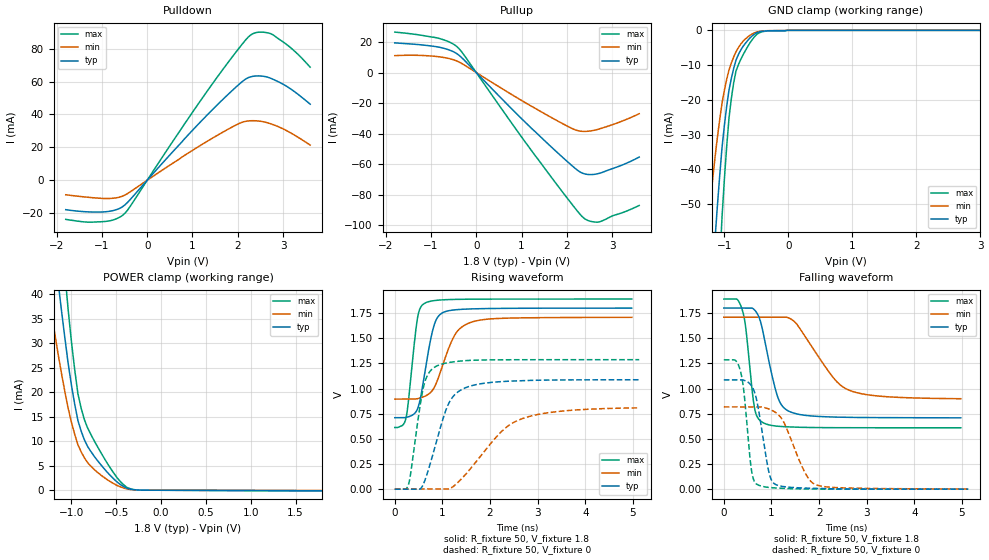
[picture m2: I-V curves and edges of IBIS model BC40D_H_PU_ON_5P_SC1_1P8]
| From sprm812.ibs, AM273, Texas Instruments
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|   Model Cell BC40D_H_PU_ON_5P_SC1_1P8
|BC40D_H_PU_ON_5P_SC1_1P8
[Model]   BC40D_H_PU_ON_5P_SC1_1P8
Model_type   I/O
Polarity   Non-Inverting
Enable   Active-Low
Vinl =  0.63
Vinh =  1.17
Cref =  15pF
Rref =  100.0000M
Vref =  0V
Vmeas =  0.9
C_comp   2.364487p   2.290698p   2.389419p
|[Input load] weak_pu_on
|[Output drive] slow
|[supplytol] 5
|[temp] ind
[Model Spec]
Vinl   0.63   0.5985   0.6615
Vinh   1.17   1.1115   1.2285
[Temperature Range]   25   125   -40
[Voltage Range]   1.8   1.71   1.89
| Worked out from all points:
|   slope of the pulldown table from 0 to 0.27 V, typ, clamps not added: 32.2 ohm
|   slope of the pullup table from 0 to 0.27 V, typ, clamps not added: 32.6 ohm
|   GND clamp passes 1 mA (typ) near -0.52 V on its own axis
|   POWER clamp passes 1 mA (typ) near -0.44 V on its own axis
|   rising waveform, R_fixture 50, V_fixture 1.8: 20-80 % time 249ps typ, 402ps min, 171ps max; typ from 0.71 V to 1.8 V
|   rising waveform, R_fixture 50, V_fixture 0: 20-80 % time 430ps typ, 919ps min, 246ps max; typ from 0 V to 1.09 V
|   falling waveform, R_fixture 50, V_fixture 1.8: 20-80 % time 310ps typ, 721ps min, 172ps max; typ from 1.8 V to 0.71 V
|   falling waveform, R_fixture 50, V_fixture 0: 20-80 % time 228ps typ, 434ps min, 155ps max; typ from 1.09 V to 0.002 V
| Nom Voltages:
|   VDD=1.1, VDDS=1.8, VDDS18=1.8, ESD_BIASFET=0, VSS=0, VSSS=0
| Min Voltages:
|   VDD=1.045, VDDS=1.71, VDDS18=1.71, ESD_BIASFET=0, VSS=0, VSSS=0
| Max Voltages:
|   VDD=1.16, VDDS=1.89, VDDS18=1.89, ESD_BIASFET=0, VSS=0, VSSS=0
[POWER_clamp]
|   voltage   I(typ)   I(min)   I(max)
-1.8V     158.8mA    112.5mA    219.8mA
-1.255V   59.97mA    40.01mA    84.91mA
-1.145V   41.92mA    27.41mA    59.76mA
-1.109V   36.32mA    23.62mA    51.83mA
-1.073V   30.96mA    20.04mA    44.16mA
-1.036V   25.83mA    16.67mA    36.76mA
-963.6mV  17.54mA    11.39mA    24.56mA
-890.9mV  12.01mA    7.798mA    16.67mA
-818.2mV  8.875mA    5.598mA    12.64mA
-563.6mV  2.954mA    1.726mA    4.46mA
-272.7mV  55.97uA    39.54uA    57.56uA
1.8V      -99.94uA   -59.14uA   -145.1uA
[Pulldown]
|   voltage   I(typ)   I(min)   I(max)
-1.8V     -17.92mA   -8.85mA    -23.8mA
-1.309V   -19.26mA   -10.37mA   -25.51mA
-927.3mV  -19.22mA   -11.12mA   -25.08mA
-654.5mV  -17.65mA   -10.56mA   -23.13mA
-490.9mV  -14.97mA   -8.985mA   -20.05mA
1.364V    40.78mA    24.32mA    55.7mA
2.073V    59.41mA    35mA       81.9mA
2.291V    62.96mA    36.2mA     88.48mA
2.509V    63.41mA    35.84mA    90.12mA
2.782V    61.38mA    33.82mA    88.42mA
3.218V    54.59mA    28.02mA    79.45mA
3.6V      46.26mA    21.39mA    68.79mA
[Pullup]
|   voltage   I(typ)   I(min)   I(max)
-1.8V     19.42mA    11.07mA    26.5mA
-818.2mV  16.58mA    10.3mA     22.34mA
-545.5mV  14.19mA    8.748mA    19.29mA
-381.8mV  11.34mA    6.915mA    15.7mA
1.255V    -37.51mA   -22.64mA   -52.53mA
2.127V    -61.34mA   -36.82mA   -86.78mA
2.291V    -65.12mA   -38.38mA   -92.82mA
2.4V      -66.46mA   -38.59mA   -95.91mA
2.564V    -66.86mA   -38.08mA   -97.75mA
2.727V    -65.99mA   -36.9mA    -97.78mA
3.273V    -60.01mA   -31.26mA   -91.34mA
3.6V      -55.4mA    -26.98mA   -87.12mA
[GND_clamp]
|   voltage   I(typ)   I(min)   I(max)
-1.8V     -270.2mA   -170.2mA   -430.1mA
-1.255V   -91.68mA   -55.92mA   -148.5mA
-1.145V   -59.94mA   -36.46mA   -97.14mA
-1.109V   -50.51mA   -30.84mA   -81.61mA
-1.073V   -41.77mA   -25.67mA   -67.13mA
-1.036V   -33.71mA   -20.95mA   -53.68mA
-927.3mV  -17.15mA   -11.38mA   -25.19mA
-854.5mV  -10.96mA   -7.663mA   -15.08mA
-781.8mV  -7.031mA   -5.001mA   -9.947mA
-563.6mV  -1.569mA   -1.041mA   -2.641mA
-18.18mV  0A         0A         0A
3.6V      0A         0A         0A
[Ramp]
| variable   typ   min   max
dV/dt_f 0.66084492/0.31281459n 0.49606735/0.73709622n 0.77242944/0.17411475n
dV/dt_r  0.6586843/0.43252322n 0.50244453/0.96261999n 0.77697469/0.24742763n
R_load = 50
[Rising Waveform]
R_fixture = 50
V_fixture = 1.8
V_fixture_min = 1.71
V_fixture_max = 1.89
|   time   V(typ)   V(min)   V(max)
0s        710.5mV    895.2mV    613.1mV
234.3ps   712.4mV    895.2mV    704.9mV
473.9ps   794.1mV    899.3mV    1.692V
535.4ps   896.2mV    907mV      1.802V
630.8ps   1.159V     923.5mV    1.849V
779.8ps   1.548V     976mV      1.871V
900.3ps   1.709V     1.088V     1.879V
1.259ns   1.783V     1.532V     1.887V
1.579ns   1.792V     1.655V     1.889V
4.974ns   1.8V       1.708V     1.89V
[Rising Waveform]
R_fixture = 50
V_fixture = 0
V_fixture_min = 0
V_fixture_max = 0
|   time   V(typ)   V(min)   V(max)
0s        0V         2.16mV     2.755mV
285.8ps   0V         2.16mV     42.71mV
600.7ps   49.88mV    2.16mV     1.012V
703.9ps   189.4mV    2.16mV     1.147V
867.5ps   461mV      2.16mV     1.221V
1.161ns   878.2mV    5.785mV    1.261V
1.558ns   1.021V     185.9mV    1.28V
2.241ns   1.069V     573.1mV    1.286V
2.669ns   1.079V     700mV      1.287V
5.131ns   1.088V     808.1mV    1.287V
[Falling Waveform]
R_fixture = 50
V_fixture = 1.8
V_fixture_min = 1.71
V_fixture_max = 1.89
|   time   V(typ)   V(min)   V(max)
0s        1.801V     1.71V      1.89V
275.2ps   1.801V     1.71V      1.89V
381.3ps   1.801V     1.71V      1.792V
462.6ps   1.801V     1.71V      1.598V
642.2ps   1.783V     1.71V      815.5mV
820.2ps   1.569V     1.71V      663.4mV
1.125ns   927.1mV    1.71V      627.2mV
1.384ns   771.8mV    1.697V     619.6mV
2.587ns   715.3mV    994.2mV    612.1mV
4.974ns   710.2mV    900.2mV    611.7mV
[Falling Waveform]
R_fixture = 50
V_fixture = 0
V_fixture_min = 0
V_fixture_max = 0
|   time   V(typ)   V(min)   V(max)
0s        1.087V     819.1mV    1.286V
345.5ps   1.087V     819.1mV    1.182V
422ps     1.083V     819.1mV    970.7mV
577.5ps   1.031V     819.1mV    201.7mV
709.7ps   841.6mV    819.1mV    46.24mV
946.7ps   170.7mV    797.9mV    19.34mV
1.111ns   43.82mV    755.1mV    13.4mV
1.723ns   12.57mV    150.1mV    3.96mV
1.938ns   9.816mV    45.11mV    3.227mV
5.131ns   2.077mV    3.497mV    2.429mV
